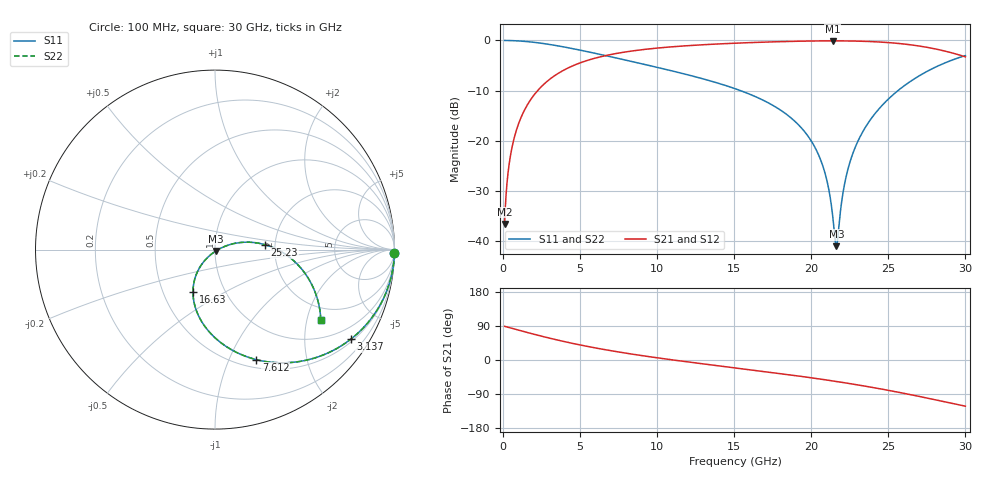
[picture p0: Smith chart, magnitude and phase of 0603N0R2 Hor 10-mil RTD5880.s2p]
# GHz S MA R 50
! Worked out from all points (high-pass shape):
!   3201 points, 100 MHz to 30 GHz, reference 50 ohm
!   highest |S21| = -0.08 dB at 21.4 GHz (marker M1); lowest = -36.6 dB at 100 MHz (marker M2)
!   |S21| within 3 dB of the highest: 6.568 GHz to 29.81 GHz (23.24 GHz wide, 128 % of centre)
!   lowest |S11| = -41.0 dB at 21.63 GHz (marker M3), VSWR 1.02, Z = 50.5 - j0.754 ohm
!   |S11| at or under -10 dB: 15.41 GHz to 25.62 GHz (10.22 GHz wide, 49.8 % of centre)
!   |S22| runs from -41.0 to 0.0 dB; largest |S21 - S12| = 0
!   S11 on the Smith chart (normalised r, x): 100 MHz: open; 3.137 GHz: 0.58, -3.23; 7.612 GHz: 0.59, -1.27; 16.63 GHz: 0.71, -0.36; 25.23 GHz: 1.77, +0.10; 30 GHz: 1.56, -2.43
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0.1  0.9999 -1.1  0.01485 88.9  0.01485 88.9  0.9999 -1.1
0.4550625  0.9977 -5.1  0.06745 84.9  0.06745 84.9  0.9977 -5.1
0.9783125  0.9896 -10.9  0.1438 79.1  0.1438 79.1  0.9896 -10.9
1.856625  0.9639 -20.5  0.266 69.5  0.266 69.5  0.9639 -20.5
3.136719  0.9059 -33.5  0.4227 56.5  0.4227 56.5  0.9059 -33.5
5.089563  0.7955 -51.0  0.6046 39.0  0.6046 39.0  0.7955 -51.0
7.612375  0.6547 -69.4  0.7538 20.4  0.7538 20.4  0.6547 -69.4
10.06978  0.5362 -84.3  0.8412 5.4  0.8412 5.4  0.5362 -84.3
15.05  0.3309 -109.9  0.939 -20.7  0.939 -20.7  0.3309 -109.9
16.62909  0.2646 -117.6  0.9589 -28.7  0.9589 -28.7  0.2646 -117.6
18.66603  0.17 -127.3  0.9787 -39.5  0.9787 -39.5  0.17 -127.3
20.03956  0.09725 -132.7  0.9875 -47.2  0.9875 -47.2  0.09725 -132.7
20.89919  0.04709 -132.1  0.9904 -52.2  0.9904 -52.2  0.04709 -132.1
21.40375  0.01704 -114.6  0.9909 -55.3  0.9909 -55.3  0.01704 -114.6
21.628  0.008909 -57.0  0.9908 -56.7  0.9908 -56.7  0.008909 -57.0
22.16994  0.03781 15.4  0.9896 -60.1  0.9896 -60.1  0.03781 15.4
22.73056  0.07726 18.7  0.9867 -63.8  0.9867 -63.8  0.07726 18.7
23.67428  0.1492 15.4  0.9774 -70.3  0.9774 -70.3  0.1492 15.4
25.01978  0.2622 7.0  0.9519 -80.2  0.9519 -80.2  0.2622 7.0
25.22534  0.2804 5.6  0.9465 -81.8  0.9465 -81.8  0.2804 5.6
27.40244  0.4814 -11.4  0.8599 -99.5  0.8599 -99.5  0.4814 -11.4
30  0.7072 -33.5  0.6864 -121.9  0.6864 -121.9  0.7072 -33.5
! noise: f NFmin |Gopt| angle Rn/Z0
0.1  0.0009163  0.9853  1.045  0.01426
3.417  0.00357  0.7977  12.3  0.003612
6.743  0.005982  0.7595  20.38  0.004884
10.06  0.008377  0.7449  28.62  0.006203
13.39  0.011  0.7427  36.85  0.007739
16.7  0.01407  0.7497  44.94  0.009702
20.03  0.01793  0.7645  52.9  0.01245
23.35  0.02309  0.7865  60.7  0.01664
26.67  0.03057  0.8151  68.42  0.02375
30  0.0426  0.8501  76.08  0.03771
